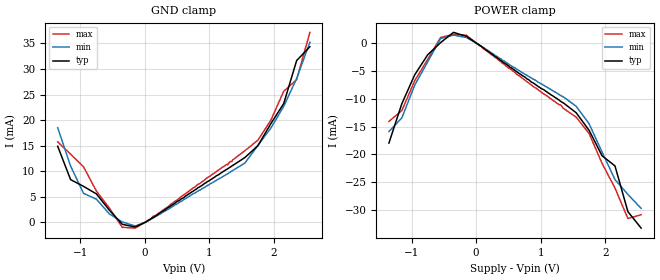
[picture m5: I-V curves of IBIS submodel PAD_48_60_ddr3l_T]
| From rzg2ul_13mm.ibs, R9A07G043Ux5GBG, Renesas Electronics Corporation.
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[Submodel]  PAD_48_60_ddr3l_T
Submodel_type Dynamic_clamp
[GND Clamp]
| Voltage   I(typ)   I(min)   I(max)
-1.35V    14.9mA     18.52mA    15.75mA
-1.15V    8.374mA    11.02mA    13.35mA
-950mV    7.058mA    5.693mA    10.89mA
-750mV    5.572mA    4.541mA    6.109mA
-350mV    -360.4uA   99.84uA    -943.8uA
-150mV    -888.9uA   -699.8uA   -1.111mA
1.55V     12.7mA     11.62mA    14.04mA
1.75V     15.01mA    15.06mA    16.08mA
1.95V     19.31mA    18.43mA    19.98mA
2.15V     23.25mA    22.7mA     25.65mA
2.35V     31.65mA    28.16mA    27.91mA
2.555V    34.35mA    35.24mA    37.16mA
[POWER Clamp]
| Voltage   I(typ)   I(min)   I(max)
-1.35V    -17.96mA   -15.91mA   -14.08mA
-1.15V    -10.9mA    -13.45mA   -12.13mA
-750mV    -2.133mA   -3.406mA   -2.959mA
-550mV    48.89uA    780.2uA    978.6uA
-350mV    1.887mA    1.401mA    1.523mA
-150mV    1.17mA     955.6uA    1.367mA
1.55V     -12.54mA   -11.39mA   -13.33mA
1.75V     -15.7mA    -14.52mA   -16.27mA
1.95V     -20.25mA   -19.58mA   -21.62mA
2.15V     -22.07mA   -24.52mA   -26.04mA
2.35V     -30.27mA   -27.18mA   -31.51mA
2.555V    -33.23mA   -29.69mA   -30.82mA
